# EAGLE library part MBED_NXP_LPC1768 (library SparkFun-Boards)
mbed LPC1768 board footprint Boards using this footprint: mbed - LPC1768 (Cortex-M3) (DEV-09564)
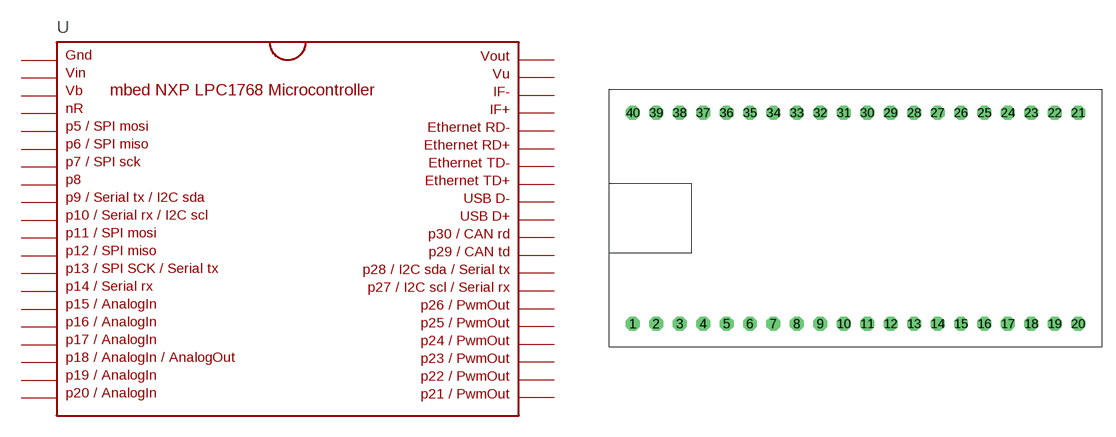
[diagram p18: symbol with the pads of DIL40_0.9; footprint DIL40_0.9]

Designator prefix -

## MBED_NXP_LPC1768 (PROD_ID: COMP-12167; VALUE: MBED1768)  [DIL40_0.9]
1  P$1
2  P$2
3  P$3
4  P$4
5  P$5
6  P$6
7  P$7
8  P$8
9  P$9
10  P$10
11  P$11
12  P$12
13  P$13
14  P$14
15  P$15
16  P$16
17  P$17
18  P$18
19  P$19
20  P$20
21  P$21
22  P$22
23  P$23
24  P$24
25  P$25
26  P$26
27  P$27
28  P$28
29  P$29
30  P$30
31  P$31
32  P$32
33  P$33
34  P$34
35  P$35
36  P$36
37  P$37
38  P$38
39  P$39
40  P$40

## Footprint DIL40_0.9 (pad centres in mm)
Dual inline 40 pin package for mbed microcontroller development platform.
drill 1 pad 1.397 octagon: 1 -22.86,-11.43; 2 -20.32,-11.43; 3 -17.78,-11.43; 4 -15.24,-11.43; 5 -12.7,-11.43; 6 -10.16,-11.43; 7 -7.62,-11.43; 8 -5.08,-11.43; 9 -2.54,-11.43; 10 0,-11.43; 11 2.54,-11.43; 12 5.08,-11.43; 13 7.62,-11.43; 14 10.16,-11.43; 15 12.7,-11.43; 16 15.24,-11.43; 17 17.78,-11.43; 18 20.32,-11.43; 19 22.86,-11.43; 20 25.4,-11.43; 21 25.4,11.43; 22 22.86,11.43; 23 20.32,11.43; 24 17.78,11.43; 25 15.24,11.43; 26 12.7,11.43; 27 10.16,11.43; 28 7.62,11.43; 29 5.08,11.43; 30 2.54,11.43; 31 0,11.43; 32 -2.54,11.43; 33 -5.08,11.43; 34 -7.62,11.43; 35 -10.16,11.43; 36 -12.7,11.43; 37 -15.24,11.43; 38 -17.78,11.43; 39 -20.32,11.43; 40 -22.86,11.43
